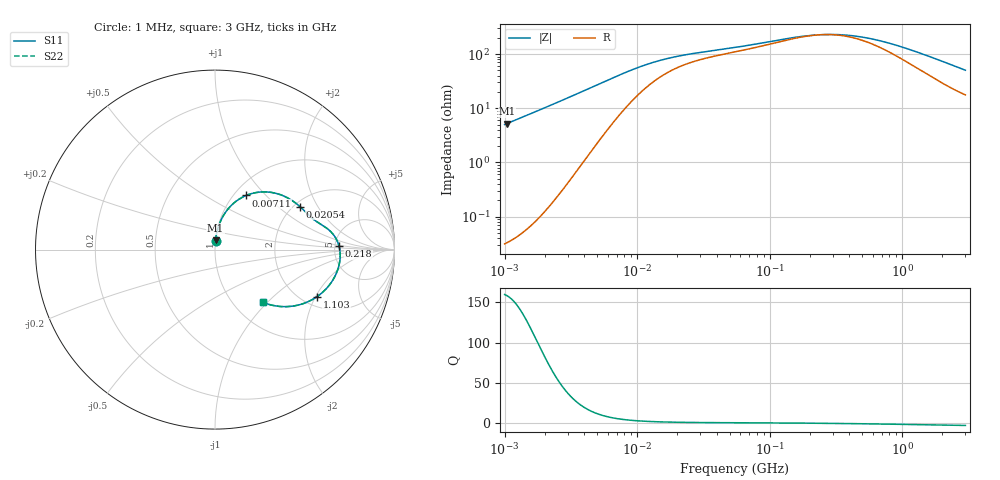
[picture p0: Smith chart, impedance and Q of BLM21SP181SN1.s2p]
! BLM21SP181SN1
# Hz S RI R 50
!Freq.(Hz) S11(Real) S11(Imag) S21(Real) S21(Imag) S12(Real) S12(Imag) S22(Real) S22(Imag)
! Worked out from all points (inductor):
!   401 points, 1 MHz to 3 GHz, reference 50 ohm
!   read as one part in series: L = 800 nH near 1.041 MHz
!   highest Q = 158 at 1.041 MHz (marker M1), where L = 798 nH
!   self-resonance near 247.7 MHz
!   S11 on the Smith chart (normalised r, x): 1 MHz: 1.00, +0.10; 7.11 MHz: 1.14, +0.78; 20.54 MHz: 2.15, +1.43; 218 MHz: 5.46, +0.38; 1.103 GHz: 2.39, -2.06; 3 GHz: 1.35, -0.94
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1000000  0.00282 0.0499  0.9972 -0.0499  0.9972 -0.0499  0.00282 0.0499
1040844  0.00304 0.052  0.997 -0.052  0.997 -0.052  0.00304 0.052
2097170  0.0126 0.1053  0.9874 -0.1053  0.9874 -0.1053  0.0126 0.1053
3823119  0.0473 0.1905  0.9527 -0.1905  0.9527 -0.1905  0.0473 0.1905
5266264  0.096 0.2513  0.904 -0.2513  0.904 -0.2513  0.096 0.2513
7110411  0.1743 0.3019  0.8257 -0.3019  0.8257 -0.3019  0.1743 0.3019
9992459  0.2906 0.3212  0.7094 -0.3212  0.7094 -0.3212  0.2906 0.3212
1.461624e7  0.4063 0.2873  0.5937 -0.2873  0.5937 -0.2873  0.4063 0.2873
2.054061e7  0.4736 0.2393  0.5264 -0.2393  0.5264 -0.2393  0.4736 0.2393
3.190472e7  0.5262 0.1885  0.4738 -0.1885  0.4738 -0.1885  0.5262 0.1885
5.477226e7  0.576 0.1497  0.424 -0.1497  0.424 -0.1497  0.576 0.1497
1.103592e8  0.6454 0.0995  0.3546 -0.0995  0.3546 -0.0995  0.6454 0.0995
2.094008e8  0.6899 0.0238  0.3101 -0.0238  0.3101 -0.0238  0.6899 0.0238
2.179536e8  0.6914 0.0183  0.3086 -0.0183  0.3086 -0.0183  0.6914 0.0183
3.002264e8  0.6975 -0.0289  0.3025 0.0289  0.3025 0.0289  0.6975 -0.0289
4.0536e8  0.693 -0.0774  0.307 0.0774  0.307 0.0774  0.693 -0.0774
5.583748e8  0.675 -0.1343  0.325 0.1343  0.325 0.1343  0.675 -0.1343
8.005644e8  0.6328 -0.203  0.3672 0.203  0.3672 0.203  0.6328 -0.203
1.10276e9  0.5697 -0.2614  0.4303 0.2614  0.4303 0.2614  0.5697 -0.2614
1.818868e9  0.424 -0.316  0.576 0.316  0.576 0.316  0.424 -0.316
2.312676e9  0.3457 -0.3149  0.6543 0.3149  0.6543 0.3149  0.3457 -0.3149
3e9  0.2676 -0.2937  0.7324 0.2937  0.7324 0.2937  0.2676 -0.2937
